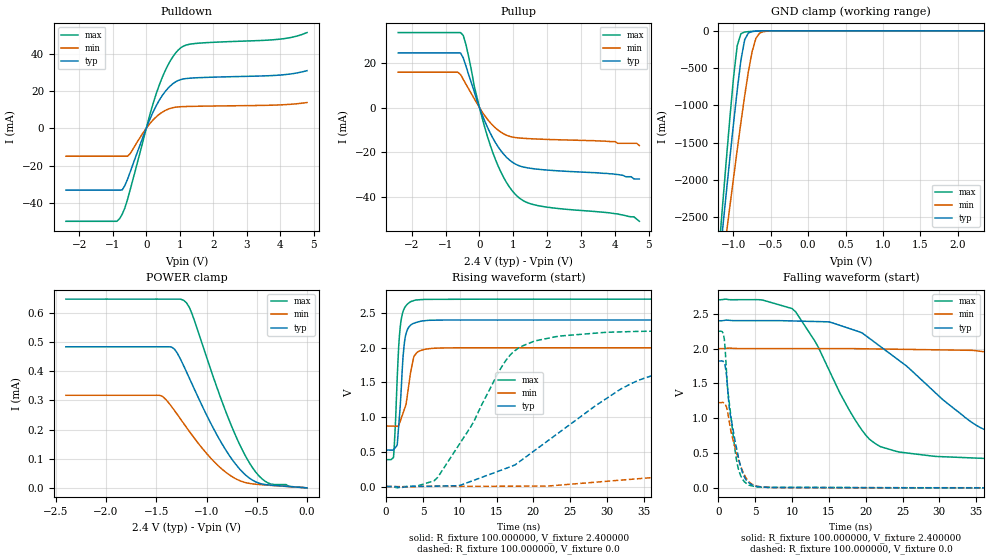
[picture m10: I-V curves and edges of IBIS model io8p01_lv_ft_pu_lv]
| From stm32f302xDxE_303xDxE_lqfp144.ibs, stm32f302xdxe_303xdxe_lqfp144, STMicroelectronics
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|   Model io8p01_lv_ft_pu_lv
[Model]  io8p01_lv_ft_pu_lv
Model_type I/O
Polarity   Non-Inverting
Enable   Active-Low
Vinl =   0.720000V
Vinh =   1.680000V
Vmeas =  1.200000V
Cref =   50.000000pF
Rref =   100.000000M
Vref =   0.0V
C_comp   5.024800pF   4.846300pF   5.260300pF
[Temperature Range]   25.000000   0.125000k   -40.000000
[Pullup Reference]   2.400000V   2.000000V   2.700000V
[Pulldown Reference]   0.0V   0.0V   0.0V
[POWER Clamp Reference]   2.400000V   2.000000V   2.700000V
[GND Clamp Reference]   0.0V   0.0V   0.0V
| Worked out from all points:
|   slope of the pulldown table from 0 to 0.36 V, typ, clamps not added: 25.5 ohm
|   slope of the pullup table from 0 to 0.36 V, typ, clamps not added: 28.4 ohm
|   GND clamp passes 1 mA (typ) near -0.60 V on its own axis
|   rising waveform, R_fixture 100.000000, V_fixture 2.400000: 20-80 % time 711ps typ, 1.14ns min, 628ps max; typ from 0.527 V to 2.4 V
|   rising waveform, R_fixture 100.000000, V_fixture 0.0: 20-80 % time 14.6ns typ, 42.7ns min, 7.2ns max; typ from 0.001 V to 1.82 V
|   falling waveform, R_fixture 100.000000, V_fixture 2.400000: 20-80 % time 12.9ns typ, 32.5ns min, 7.07ns max; typ from 2.4 V to 0.527 V
|   falling waveform, R_fixture 100.000000, V_fixture 0.0: 20-80 % time 1.65ns typ, 1.85ns min, 1.36ns max; typ from 1.82 V to 0.001 V
[Pulldown]
|Voltage   I(typ)   I(min)   I(max)
-2.4V     -33.16mA   -14.98mA   -49.86mA
-880mV    -33.16mA   -14.98mA   -49.86mA
-800mV    -33.16mA   -14.98mA   -48.55mA
-640mV    -30.75mA   -14.98mA   -42.77mA
-480mV    -23.43mA   -13.57mA   -32.92mA
80mV      3.651mA    1.905mA    5.506mA
400mV     15.37mA    7.665mA    23.73mA
720mV     22.75mA    10.69mA    36.23mA
1.04V     26.18mA    11.57mA    43.27mA
1.52V     27.09mA    11.81mA    45.55mA
4V        28.55mA    12.55mA    47.81mA
4.8V      30.9mA     13.81mA    51.31mA
[Pullup]
|Voltage   I(typ)   I(min)   I(max)
-2.4V     24.56mA    15.9mA     33.69mA
-640mV    24.56mA    15.9mA     33.69mA
-480mV    22.33mA    12.71mA    32.43mA
-400mV    18.72mA    10.52mA    28.28mA
-160mV    7.425mA    4.163mA    10.02mA
0V        80fA       15.3pA     0A
320mV     -11.51mA   -6.781mA   -16.98mA
720mV     -21mA      -11.8mA    -31.53mA
1.2V      -26.24mA   -13.65mA   -40.82mA
1.76V     -27.69mA   -14.12mA   -44.06mA
4.08V     -30mA      -16mA      -47.7mA
4.72V     -32mA      -17mA      -51mA
[GND_clamp]
|Voltage   I(typ)   I(min)   I(max)
-2.4V     -9.914A    -9.862A    -9.419A
-1.2V     -3.21A     -3.567A    -3.02A
-1.15V    -2.709A    -3.165A    -2.399A
-1.1V     -2.213A    -2.766A    -1.788A
-1.05V    -1.726A    -2.371A    -1.195A
-950mV    -800.5mA   -1.599A    -202.1mA
-900mV    -394.9mA   -1.228A    -38.17mA
-850mV    -120.2mA   -874.5mA   -15.91mA
-750mV    -9.807mA   -279.4mA   -7.273mA
-700mV    -4.736mA   -102mA     -4.51mA
-600mV    -1.032mA   -11.09mA   -922.6uA
2.35V     0A         0A         0A
[POWER_clamp]
|Voltage   I(typ)   I(min)   I(max)
-2.4V     483.6uA    317.4uA    647uA
-1.47V    483.6uA    317.4uA    647uA
-1.32V    475.8uA    265.5uA    647uA
-1.23V    420.2uA    221.9uA    643.4uA
-1.17V    375.2uA    193uA      618uA
-1.14V    352.5uA    178.9uA    592.4uA
-840mV    147.3uA    62.31uA    290.1uA
-690mV    72.45uA    27.83uA    163.1uA
-540mV    25.83uA    13.54uA    67.87uA
-450mV    13.39uA    10.74uA    31.49uA
-360mV    9.215uA    8.523uA    13uA
0V        0A         0A         0A
[Ramp]
| variable   typ   min   max
dV/dt_r  1.09263/14.61086n   0.73347/42.64348n   1.34920/7.18231n
dV/dt_f  1.12399/12.92586n   0.67623/32.50333n   1.38682/7.05279n
R_load = 100.000000
[Rising Waveform]
R_fixture= 100.000000
V_fixture= 2.400000
V_fixture_min= 2.000000
V_fixture_max= 2.700000
|time   V(typ)   V(min)   V(max)
0s        526.5mV    872.5mV    388.6mV
1.001ns   532.9mV    871.4mV    421.5mV
1.301ns   569.5mV    870.1mV    1.004V
1.502ns   598.4mV    869.4mV    1.567V
1.902ns   1.145V     938.8mV    2.288V
2.503ns   2.091V     1.123V     2.574V
3.403ns   2.332V     1.691V     2.667V
4.204ns   2.369V     1.934V     2.689V
6.306ns   2.396V     1.991V     2.697V
49.85ns   2.4V       2V         2.7V
[Rising Waveform]
R_fixture= 100.000000
V_fixture= 0.0
V_fixture_min= 0.0
V_fixture_max= 0.0
|time   V(typ)   V(min)   V(max)
0s        1.055mV    1.354mV    939.9uV
6.507ns   6.507mV    4.43mV     83.9mV
11.51ns   75.73mV    4.543mV    864.6mV
16.52ns   272mV      5.92mV     1.854V
23.52ns   781.6mV    21.66mV    2.168V
35.04ns   1.56V      120.5mV    2.237V
52.55ns   1.783V     400.7mV    2.248V
77.58ns   1.819V     854.7mV    2.25V
107.6ns   1.823V     1.136V     2.25V
249.2ns   1.822V     1.224V     2.25V
[Falling Waveform]
R_fixture= 100.000000
V_fixture= 2.400000
V_fixture_min= 2.000000
V_fixture_max= 2.700000
|time   V(typ)   V(min)   V(max)
0s        2.4V       2V         2.7V
10.01ns   2.397V     2V         2.575V
15.02ns   2.384V     2V         1.693V
20.52ns   2.146V     1.997V     698.1mV
29.53ns   1.36V      1.983V     452mV
37.04ns   800.7mV    1.943V     419.7mV
50.55ns   606.4mV    1.72V      399.1mV
76.58ns   545.4mV    1.149V     389.3mV
101.1ns   529.7mV    965mV      388.5mV
249.2ns   526.5mV    872.5mV    388.6mV
[Falling Waveform]
R_fixture= 100.000000
V_fixture= 0.0
V_fixture_min= 0.0
V_fixture_max= 0.0
|time   V(typ)   V(min)   V(max)
0s        1.822V     1.224V     2.25V
800.8ps   1.792V     1.219V     2.127V
1.101ns   1.606V     1.154V     1.646V
1.301ns   1.352V     1.055V     1.362V
1.502ns   1.117V     924.2mV    1.191V
2.503ns   543.2mV    483.6mV    369.9mV
3.303ns   208.7mV    235.5mV    120.3mV
4.104ns   75.44mV    92.11mV    40.72mV
7.107ns   6.989mV    5.602mV    8.579mV
49.85ns   1.055mV    1.354mV    939.9uV
